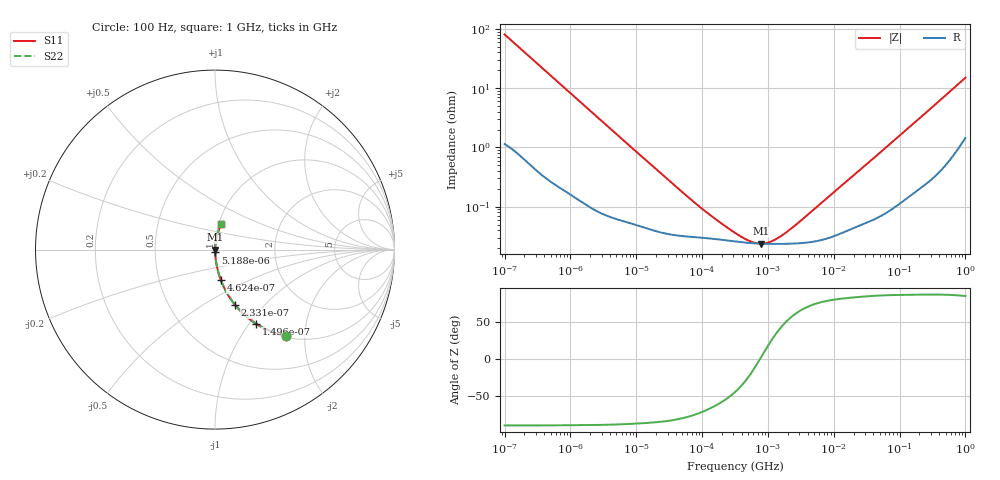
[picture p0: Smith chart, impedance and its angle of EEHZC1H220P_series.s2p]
!  *** S-Parameter ***
!  Copyright (C) Panasonic Industry
!  Conductive Polymer Hybrid Aluminum Electrolytic Capacitor
!  Parts No. EEHZC1H220P
!  Connection Mode : Series
!  1  o---||---o  2
!  GND o--------o GND
!  Conditions : Temperature = 20 degC , DC Bias = 0 V
! Frequency Range : 100Hz  -  1GHz  [ 401 Steps ]
# Hz S RI R 50
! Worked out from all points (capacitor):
!   401 points, 100 Hz to 1 GHz, reference 50 ohm
!   read as one part in series: C = 19.7 uF near 108.4 Hz
!   lowest |Z| = 23.8 mohm at 798.9 kHz (marker M1)
!   series resonance near 759.4 kHz, so ESL is about 2.2 nH
!   S11 on the Smith chart (normalised r, x): 100 Hz: 1.02, -1.61; 149.6 Hz: 1.02, -1.08; 233.1 Hz: 1.01, -0.70; 462.4 Hz: 1.01, -0.35; 5.188 kHz: 1.00, -0.03; 1 GHz: 1.03, +0.30
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100  0.3945 -0.4817  0.6055 0.4817  0.6055 0.4817  0.3945 -0.4817
149.6236  0.2295 -0.413  0.7705 0.413  0.7705 0.413  0.2295 -0.413
233.0773  0.1121 -0.3079  0.8879 0.3079  0.8879 0.3079  0.1121 -0.3079
321.7363  0.0635 -0.2363  0.9365 0.2363  0.9365 0.2363  0.0635 -0.2363
462.381  0.0328 -0.1704  0.9672 0.1704  0.9672 0.1704  0.0328 -0.1704
780.7284  0.0128 -0.1036  0.9872 0.1036  0.9872 0.1036  0.0128 -0.1036
1487.647  0.00426 -0.0552  0.9957 0.0552  0.9957 0.0552  0.00426 -0.0552
5188  0.000868 -0.0161  0.9991 0.0161  0.9991 0.0161  0.000868 -0.0161
22130.95  0.000389 -0.00387  0.9996 0.00387  0.9996 0.00387  0.000389 -0.00387
98287.89  0.0003 -0.000889  0.9997 0.000889  0.9997 0.000889  0.0003 -0.000889
316227.8  0.000258 -0.000253  0.9997 0.000253  0.9997 0.000253  0.000258 -0.000253
533949.3  0.000244 -9.47e-05  0.9998 9.47e-05  0.9998 9.47e-05  0.000244 -9.47e-05
653130.6  0.00024 -4.01e-05  0.9998 4.01e-05  0.9998 4.01e-05  0.00024 -4.01e-05
798913.9  0.000238 1.36e-05  0.9998 -1.36e-05  0.9998 -1.36e-05  0.000238 1.36e-05
1059254  0.000236 9.09e-05  0.9998 -9.09e-05  0.9998 -9.09e-05  0.000236 9.09e-05
1522299  0.000235 0.000203  0.9998 -0.000203  0.9998 -0.000203  0.000235 0.000203
2371374  0.000238 0.000377  0.9998 -0.000377  0.9998 -0.000377  0.000238 0.000377
4704354  0.000256 0.000809  0.9997 -0.000809  0.9997 -0.000809  0.000256 0.000809
6.99842e7  0.000971 0.0111  0.999 -0.0111  0.999 -0.0111  0.000971 0.0111
3.235937e8  0.00542 0.0488  0.9946 -0.0488  0.9946 -0.0488  0.00542 0.0488
9.225714e8  0.0303 0.1319  0.9697 -0.1319  0.9697 -0.1319  0.0303 0.1319
1e9  0.035 0.1417  0.965 -0.1417  0.965 -0.1417  0.035 0.1417
